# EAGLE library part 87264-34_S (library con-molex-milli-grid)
RECEPTACAL
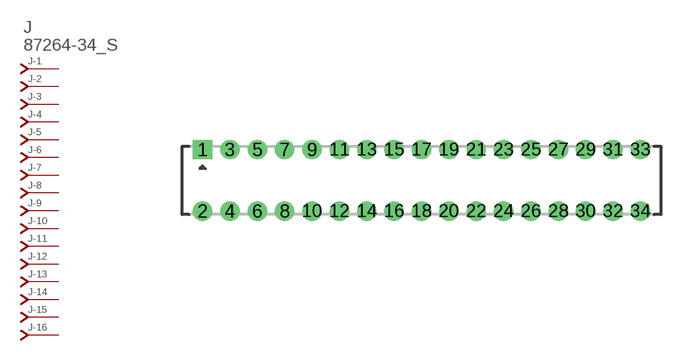
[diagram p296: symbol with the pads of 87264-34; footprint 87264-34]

Designator prefix J; gates -1=J-NV -2=J-N -3=J-N -4=J-N -5=J-N -6=J-N -7=J-N -8=J-N -9=J-N -10=J-N -11=J-N -12=J-N -13=J-N -14=J-N -15=J-N -16=J-N -17=J-N -18=J-N -19=J-N -20=J-N -21=J-N -22=J-N -23=J-N -24=J-N -25=J-N -26=J-N -27=J-N -28=J-N -29=J-N -30=J-N -31=J-N -32=J-N -33=J-N -34=J-N

## 87264-34_S  [87264-34]
1  -1:J  pas
2  -2:J  pas
3  -3:J  pas
4  -4:J  pas
5  -5:J  pas
6  -6:J  pas
7  -7:J  pas
8  -8:J  pas
9  -9:J  pas
10  -10:J  pas
11  -11:J  pas
12  -12:J  pas
13  -13:J  pas
14  -14:J  pas
15  -15:J  pas
16  -16:J  pas
17  -17:J  pas
18  -18:J  pas
19  -19:J  pas
20  -20:J  pas
21  -21:J  pas
22  -22:J  pas
23  -23:J  pas
24  -24:J  pas
25  -25:J  pas
26  -26:J  pas
27  -27:J  pas
28  -28:J  pas
29  -29:J  pas
30  -30:J  pas
31  -31:J  pas
32  -32:J  pas
33  -33:J  pas
34  -34:J  pas

## Footprint 87264-34 (pad centres in mm)
RECEPTACAL Dual Row, Side Entry
drill 0.914 square: 1 -16,2.25
drill 0.914: 2 -16,-2.25; 3 -14,2.25; 4 -14,-2.25; 5 -12,2.25; 6 -12,-2.25; 7 -10,2.25; 8 -10,-2.25; 9 -8,2.25; 10 -8,-2.25; 11 -6,2.25; 12 -6,-2.25; 13 -4,2.25; 14 -4,-2.25; 15 -2,2.25; 16 -2,-2.25; 17 0,2.25; 18 0,-2.25; 19 2,2.25; 20 2,-2.25; 21 4,2.25; 22 4,-2.25; 23 6,2.25; 24 6,-2.25; 25 8,2.25; 26 8,-2.25; 27 10,2.25; 28 10,-2.25; 29 12,2.25; 30 12,-2.25; 31 14,2.25; 32 14,-2.25; 33 16,2.25; 34 16,-2.25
